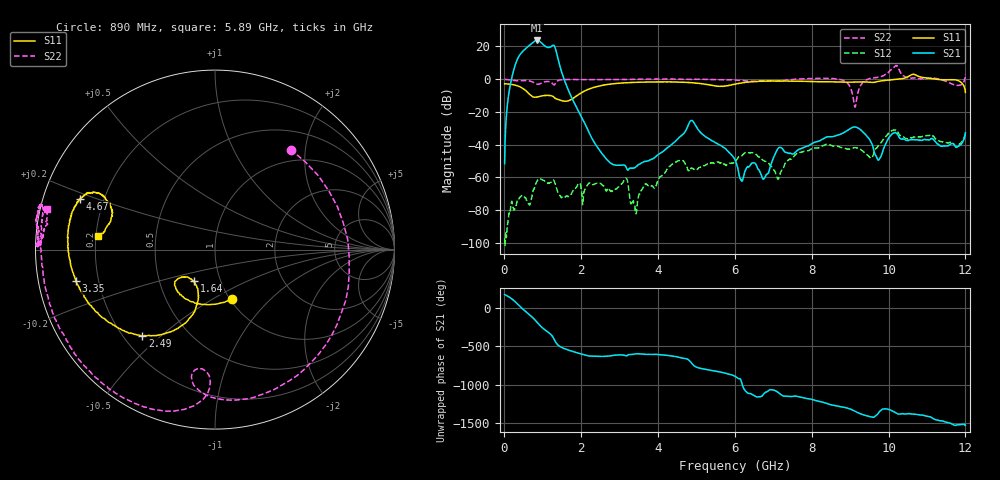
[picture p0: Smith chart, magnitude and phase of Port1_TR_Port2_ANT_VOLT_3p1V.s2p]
! Created Mon Aug 25 10:53:47 2025
# hz S ma R 50
! 2 Port Network Data from SP1.SP block
! freq  magS11  angS11  magS21  angS21  magS12  angS12  magS22  angS22
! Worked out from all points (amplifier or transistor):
!   1200 points, 10 MHz to 12 GHz, reference 50 ohm
!   highest |S21| = 23.7 dB at 860 MHz (marker M1)
!   |S21| within 3 dB of that: 654.6 MHz to 1.039 GHz (383.9 MHz wide, 45.4 % of centre)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
!   unconditionally stable (mu >= 1): start of sweep to 3.537 GHz; 4.514 GHz to 7.627 GHz; 8.679 GHz to 9.465 GHz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
!   at 2.01 GHz: K = 930.71, MAG = -10.4 dB, |S12| = -68.0 dB
!   at 6.01 GHz: K = 3076.01, MAG = -37.3 dB, |S12| = -50.6 dB
!   at 12 GHz: K = -786.00, MSG = -0.2 dB, |S12| = -32.3 dB
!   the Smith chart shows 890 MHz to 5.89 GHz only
!   S11 on the Smith chart (normalised r, x): 890 MHz: 1.02, -0.61; 1.64 GHz: 0.75, -0.28; 2.49 GHz: 0.27, -0.44; 3.35 GHz: 0.12, -0.11; 4.67 GHz: 0.11, +0.18; 5.89 GHz: 0.21, +0.06
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1e7  0.7228 178.6  0.002609 172.4  1.373e-05 -108.6  0.9838 176.3
3.5e8  0.6226 126.2  4.24 46.5  0.0001926 124.1  0.8937 2.3
5.2e8  0.4852 84.4  7.823 -32.9  0.0002533 80.2  0.9061 -99.3
7.1e8  0.3084 8.0  12.25 -113.8  0.0002259 127.4  0.8451 -179.0
8e8  0.2798 -34.9  14.59 -158.3  0.0005443 113.7  0.7552 127.9
8.6e8  0.2847 -60.5  15.24 168.4  0.0007872 90.4  0.7017 79.4
8.9e8  0.2906 -70.9  14.98 151.3  0.0008628 76.1  0.6996 52.8
1.01e9  0.312 -102.2  11.58 91.9  0.0008251 31.3  0.7979 -31.5
1.22e9  0.3116 -132.6  9.894 8.8  0.0007203 -25.0  0.7969 -95.8
1.33e9  0.2592 -141.6  8.797 -80.2  0.0006098 -111.2  0.7372 -92.0
1.41e9  0.2392 -139.9  3.712 -130.3  0.0003211 -157.4  0.9162 -102.5
1.64e9  0.2127 -123.7  0.5551 173.7  0.0002662 141.3  0.9758 -127.5
2.01e9  0.3843 -109.0  0.06848 117.6  0.0003996 58.5  0.9697 -151.6
2.49e9  0.6288 -130.1  0.006509 86.8  0.0006591 58.2  0.968 -174.8
3.35e9  0.7945 -167.3  0.001919 112.7  0.0001845 10.3  0.9864 166.2
4.01e9  0.8245 173.0  0.005013 110.9  0.0008519 75.4  1.01 167.5
4.67e9  0.8031 159.4  0.02164 60.9  0.003094 -22.1  0.9929 174.5
5.89e9  0.6557 173.3  0.005205 -149.9  0.002684 -15.6  0.9608 166.2
6.01e9  0.7043 175.8  0.003332 -175.0  0.002941 -7.3  0.9383 159.6
8.01e9  0.8441 159.5  0.01081 -114.6  0.007529 -93.3  1.042 56.5
1.001e10  0.9385 127.9  0.01629 113.3  0.02261 133.0  1.672 137.5
1.2e10  0.3912 75.5  0.02296 -93.4  0.02417 -84.4  1.424 64.9
